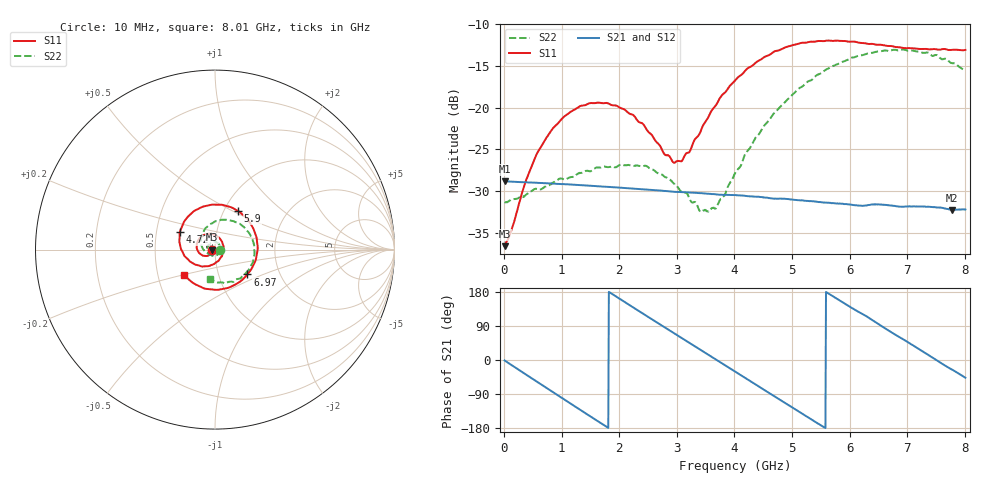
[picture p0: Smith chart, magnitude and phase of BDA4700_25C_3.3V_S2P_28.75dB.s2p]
!Agilent Technologies,E5071B,MY42404982,A.09.10
!Date: Mon Oct 20 18:15:09 2025
!Data & Calibration Information:
!Freq	S11:SOLT2(ON)	S21:SOLT2(ON)	S12:SOLT2(ON)	S22:SOLT2(ON)
# Hz S RI R 50
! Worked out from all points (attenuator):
!   801 points, 10 MHz to 8.01 GHz, reference 50 ohm
!   highest |S21| = -28.79 dB at 20 MHz (marker M1); lowest = -32.2 dB at 7.78 GHz (marker M2)
!   lowest |S11| = -36.6 dB at 10 MHz (marker M3), VSWR 1.03, Z = 48.5 - j0.123 ohm
!   |S11| at or under -10 dB: start of sweep to end of sweep
!   |S22| runs from -32.5 to -13.0 dB; largest |S21 - S12| = 0.00042
!   S11 on the Smith chart (normalised r, x): 10 MHz: 0.97, -0.00; 4.72 GHz: 0.66, +0.13; 5.9 GHz: 1.17, +0.53; 6.97 GHz: 1.37, -0.40; 8.01 GHz: 0.68, -0.20
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1e7  -0.0148 -0.00127  0.0363 -0.000791  0.0363 -0.000785  0.0272 -0.000806
2e7  -0.0151 -0.00199  0.0363 -0.00134  0.0363 -0.00143  0.0271 -0.00107
3.8e8  -0.0255 -0.0261  0.0281 -0.0221  0.028 -0.0222  0.0221 -0.0204
5.9e8  -0.0418 -0.0352  0.0182 -0.0304  0.0182 -0.0305  0.0139 -0.0295
1e9  -0.0819 -0.0246  -0.00588 -0.0344  -0.00584 -0.0344  -0.0145 -0.0347
1.35e9  -0.1024 0.0112  -0.0239 -0.0247  -0.0239 -0.0247  -0.0364 -0.0183
2.07e9  -0.0461 0.0867  -0.0301 0.0137  -0.0301 0.0137  -0.031 0.0331
2.68e9  0.0374 0.0479  -0.00372 0.0317  -0.00374 0.0317  0.0127 0.0383
2.94e9  0.0469 0.00442  0.00976 0.0298  0.00981 0.0298  0.0252 0.0249
3.06e9  0.0447 -0.0169  0.0155 0.0272  0.0153 0.0273  0.0278 0.0156
3.43e9  0.0018 -0.0748  0.0279 0.0131  0.0279 0.0131  0.0201 -0.0127
3.69e9  -0.0501 -0.0922  0.0302 0.000215  0.0303 0.000114  0.00161 -0.0252
4.01e9  -0.124 -0.0757  0.0259 -0.0151  0.0259 -0.015  -0.031 -0.0258
4.72e9  -0.196 0.0969  -0.00401 -0.0283  -0.00387 -0.0283  -0.0791 0.0525
5.35e9  -0.0596 0.2412  -0.0256 -0.0103  -0.0255 -0.0104  -0.0158 0.1466
5.9e9  0.1295 0.2149  -0.023 0.0132  -0.023 0.0131  0.1066 0.1568
6.28e9  0.2169 0.1088  -0.0115 0.0233  -0.0112 0.0233  0.1841 0.0995
6.68e9  0.2305 -0.0407  0.00566 0.0254  0.00574 0.0255  0.2188 0.000639
6.97e9  0.1801 -0.1386  0.0161 0.0199  0.0162 0.0198  0.2081 -0.0765
7.41e9  0.0349 -0.221  0.0252 0.00402  0.0252 0.00404  0.1273 -0.1633
7.78e9  -0.1049 -0.1959  0.0221 -0.0105  0.0221 -0.0106  0.0259 -0.1829
8.01e9  -0.1709 -0.1414  0.0168 -0.0179  0.0169 -0.0179  -0.0296 -0.1635
